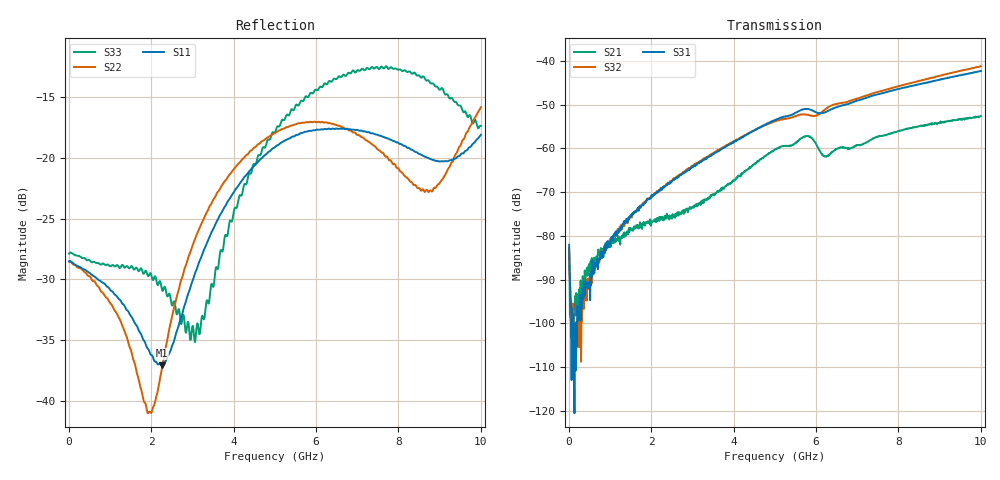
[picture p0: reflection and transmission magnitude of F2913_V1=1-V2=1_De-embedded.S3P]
! 515 Groton Road, Suite 102
! Westford, MA 01886-6024
! Device:  F2913
! Description: High Isolation SP2T RF Switch
! Frequency:  0.050 -  6.000 GHz
! Package:  4x4 mm QFN Plastic Package: 20 pin
! Ports:  3 RF, 3 DC
!  Pin  1  = GND
!  Pin  2  = GND
!  Pin  3  = RF1  =  Port 1
!  Pin  4  = GND
!  Pin  5  = GND
!  Pin  6  = GND
!  Pin  7  = GND
!  Pin  8  = RFC  =  Port 3
!  Pin  9  = GND
!  Pin 10  = GND
!  Pin 11  = GND
!  Pin 12  = GND
!  Pin 13  = RF2  =  Port 2
!  Pin 14  = GND
!  Pin 15  = GND
!  Pin 16  = C2
!  Pin 17  = C1
!  Pin 18  = GND
!  Pin 19  = GND
!  Pin 20  = Vdd
! State:  Not Recommend
! C1:  +3.3 V (Logic High)
! C2:  +3.3 V (Logic High)
! Voltage:  +3.30  Volts
! Current:  0.082 mA
! Data:  The device was measured on a F2913 evaluation board which has
!  individual transmission lines to the RF pins.  Data was collected
!  using a calibrated network analyzer.  The evaluation board was
!  de-embedded using a AFR (Keysight Technologies).
!  The reference plane is the edge of the package pin.
! Misc:
!  Action Tracker AT0430
!  WorkFront Reference Number 1053824
! Date Measured:  2018-08-23
! Date:  2018-08-24  MJV
! Note:
!  Integrated Device Technology supplies this data as a sample of measured
!  data at the package pin for this product.  Your particular data for this
!  product may vary.
!  Data was taken at 25 degrees C.
!  Integrated Device Technology reserves the right to change this data at anytime.
!Freq_(GHz)  S11M_(dB)  S11P_(deg)  S12M_(dB)  S12P_(deg)  S13M_(dB)  S13P_(deg)
!  S21M_(dB)  S21P_(deg)  S22M_(dB)  S22P_(deg)  S23M_(dB)  S23P_(deg)
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# Hz S dB R 50
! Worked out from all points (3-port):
!   1000 points, 10 MHz to 10 GHz, reference 50 ohm
!   strongest paths, dB at 10 MHz, 2.51 GHz, 5.01 GHz, 7.51 GHz, 10 GHz:
!     S31: -82.0, -67.4, -53.4, -47.6, -42.3
!     S32: -82.7, -67.4, -53.8, -47.0, -41.2
!     S21: -83.1, -75.4, -60.2, -57.3, -52.6
!   lowest |S11| = -37.1 dB at 2.26 GHz (marker M1), VSWR 1.03, Z = 49.1 + j1.07 ohm
!   |S11| at or under -10 dB: start of sweep to end of sweep
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1e7  -28.51 -179.8  -83.91 -39.9  -81.81 -36.9
     -83.13 -39.2  -28.54 -179.7  -81.93 -37.2
     -82.05 -41.6  -82.72 -39.2  -27.88 -179.3
1.09e9  -31.13 173.6  -81.04 82.0  -80.14 127.3
        -80.85 77.3  -32.40 176.2  -80.68 128.7
        -79.74 127.7  -80.04 130.3  -28.87 -153.3
1.94e9  -35.77 155.6  -77.24 81.0  -71.41 134.9
        -77.06 79.6  -40.93 127.8  -71.75 138.6
        -71.61 134.6  -71.44 137.6  -29.71 -135.9
2.26e9  -37.06 128.8  -76.50 87.4  -69.29 137.3
        -75.66 86.4  -37.36 80.2  -69.18 139.2
        -69.48 137.5  -69.09 138.0  -30.82 -131.3
3.09e9  -29.28 85.6  -73.05 101.0  -63.76 136.1
        -72.79 101.5  -26.45 69.8  -63.62 137.6
        -63.62 136.8  -63.46 137.3  -34.40 -179.9
5.01e9  -19.12 105.9  -60.32 93.3  -53.48 116.7
        -60.23 93.5  -17.95 103.2  -53.75 114.8
        -53.45 116.9  -53.78 114.8  -17.89 143.7
5.8e9  -17.84 116.0  -57.24 59.3  -50.95 96.7
       -57.13 59.8  -17.09 116.3  -52.30 101.0
       -50.96 96.7  -52.29 100.9  -15.04 151.8
6.25e9  -17.67 120.4  -61.81 55.7  -51.57 97.8
        -61.88 56.2  -17.10 122.6  -50.85 107.3
        -51.60 98.0  -50.85 107.0  -13.98 155.9
8.77e9  -20.11 106.7  -54.45 43.1  -44.70 72.2
        -54.36 42.8  -22.69 85.0  -43.89 74.1
        -44.73 72.2  -43.89 73.8  -13.86 167.9
1e10  -18.13 62.6  -52.65 23.3  -42.23 54.4
      -52.59 23.1  -15.87 39.9  -41.15 53.1
      -42.25 54.6  -41.15 53.1  -17.39 139.8
